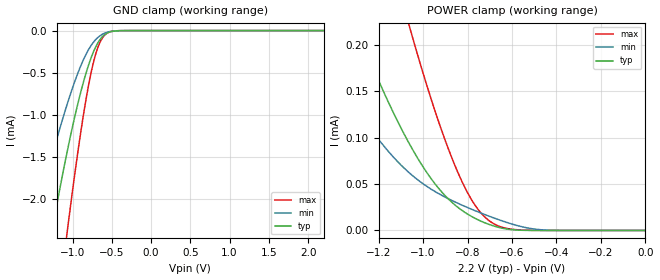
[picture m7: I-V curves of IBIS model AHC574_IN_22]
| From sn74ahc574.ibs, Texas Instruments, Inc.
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[Model]   AHC574_IN_22
Model_type  Input
Vinl = 0.5
Vinh = 1.5
| variable   typ   min   max
C_comp   1.31pF   0.83pF   1.65pF
[Temperature Range]   40   100   -40
| Ambient temperature   25   85   -40
[Voltage range]   2.2   2   2.4
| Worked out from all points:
|   GND clamp passes 1 mA (typ) near -0.97 V on its own axis
[GND Clamp]
| AHC574_IN_22
|   Voltage   I(typ)   I(min)   I(max)
-2.2V     -8.39mA    -5.403mA   -12.31mA
-1.52V    -3.837mA   -2.441mA   -6.077mA
-1.49V    -3.658mA   -2.325mA   -5.816mA
-1.27V    -2.426mA   -1.521mA   -3.962mA
-1.07V    -1.443mA   -877.8uA   -2.401mA
-920mV    -819.1uA   -474.8uA   -1.359mA
-815mV    -463.5uA   -257.2uA   -743.1uA
-725mV    -233.5uA   -127.8uA   -344uA
-630mV    -82.39uA   -49.02uA   -102.6uA
-550mV    -25.02uA   -17.18uA   -25.44uA
-425mV    -2.615uA   -1.901uA   -1.693uA
2.2V      848.6pA    557.5pA    1.495nA
[POWER Clamp]
| AHC574_IN_22
|   Voltage   I(typ)   I(min)   I(max)
-2.2V     900.8uA    580.5uA    1.555mA
-1.515V   357.1uA    219.8uA    679.6uA
-1.3V     218.5uA    131.9uA    445.7uA
-1.17V    145.5uA    89.12uA    317.4uA
-1.055V   90.53uA    60.62uA    214.5uA
-950mV    51.41uA    42.49uA    131.5uA
-865mV    29.22uA    31.69uA    74.87uA
-785mV    15.52uA    23.18uA    34.33uA
-710mV    7.127uA    16.02uA    11.88uA
-625mV    1.601uA    8.786uA    2.25uA
-470mV    19.6nA     759.5nA    55.22nA
-24.94fV  848.6pA    302.4pA    2.398nA
